DATA_BLOCK DB91
TITLE =

AUTHOR:INA
FAMILY:StateMac
NAME:nb
VERSION:00.00


    FB91


BEGIN
       Write:=FALSE
       NodeID:=B#16#00
       Done:=FALSE
       Err:=FALSE
       ErrNo:=L#0
       xEdgeMerker:=FALSE
       xEdgeFlag:=FALSE
       xStep:=0
       xFaultReset:=W#16#0080

END_DATA_BLOCK
